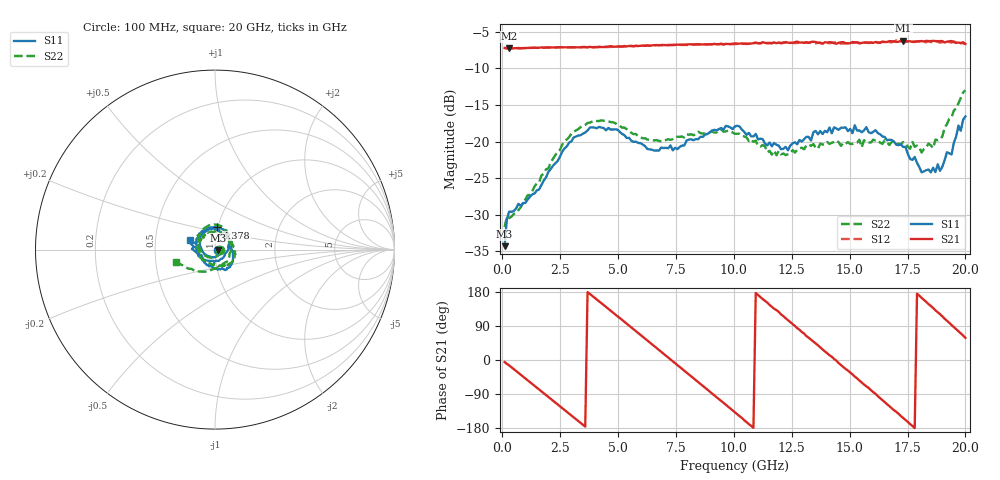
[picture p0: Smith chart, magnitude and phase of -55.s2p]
!Agilent Technologies,N5230C,MY49001569,A.09.33.09
!Agilent N5230C: A.09.33.09
!Date: Tuesday, July 28, 2015 16:40:22
!Correction: S11(Full 2 Port(1,2))
!S21(Full 2 Port(1,2))
!S12(Full 2 Port(1,2))
!S22(Full 2 Port(1,2))
!S2P File: Measurements: S11, S21, S12, S22:
# Hz S  dB  R 50
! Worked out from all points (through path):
!   201 points, 100 MHz to 20 GHz, reference 50 ohm
!   highest |S21| = -6.18 dB at 17.31 GHz (marker M1); lowest = -7.3 dB at 299 MHz (marker M2)
!   group delay of S21, straight-line fit = 141 ps
!   lowest |S11| = -34.3 dB at 100 MHz (marker M3), VSWR 1.04, Z = 52 - j0.208 ohm
!   |S11| at or under -10 dB: start of sweep to end of sweep
!   |S22| runs from -31.7 to -13.0 dB; largest |S21 - S12| = 0.02
!   S11 on the Smith chart (normalised r, x): 100 MHz: 1.04, -0.00; 4.378 GHz: 1.00, +0.25; 20 GHz: 0.75, +0.08
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1e8  -34.31 -6.0  -7.19 -5.3  -7.18 -4.8  -31.70 -5.9
2.99e8  -29.57 -18.7  -7.26 -14.4  -7.26 -14.7  -30.48 -21.7
1.891e9  -24.88 -148.2  -7.13 -92.8  -7.12 -92.6  -23.79 -148.7
3.483e9  -18.91 120.4  -7.05 -170.9  -7.09 -171.3  -17.80 124.0
4.3785e9  -18.13 83.7  -7.06 145.0  -7.06 144.8  -17.15 89.2
5.5725e9  -19.89 48.5  -6.94 86.0  -6.92 85.6  -18.80 52.2
6.7665e9  -21.24 19.5  -6.84 26.4  -6.81 26.2  -19.91 21.7
7.662e9  -20.73 0.2  -6.75 -18.3  -6.75 -18.7  -19.35 2.1
8.657e9  -19.35 -21.8  -6.72 -68.1  -6.70 -68.8  -18.90 -15.6
9.453e9  -18.14 -43.4  -6.60 -107.9  -6.67 -109.1  -18.34 -30.3
1.005e10  -17.91 -58.3  -6.57 -138.2  -6.66 -138.5  -18.93 -42.2
1.0846e10  -19.30 -80.5  -6.53 -178.8  -6.52 -179.0  -20.04 -63.9
1.1443e10  -20.52 -103.3  -6.52 151.6  -6.51 150.3  -21.46 -84.0
1.2438e10  -20.54 -152.2  -6.51 99.9  -6.47 99.1  -21.59 -125.4
1.3433e10  -18.72 162.1  -6.34 48.4  -6.54 47.9  -20.33 -167.8
1.47265e10  -18.11 124.7  -6.39 -18.3  -6.60 -18.3  -20.19 148.1
1.57215e10  -18.03 108.8  -6.44 -69.5  -6.45 -70.3  -20.16 127.1
1.67165e10  -19.74 66.5  -6.26 -121.6  -6.38 -122.2  -20.47 79.1
1.73135e10  -20.73 33.6  -6.18 -153.0  -6.28 -154.3  -20.06 42.7
1.81095e10  -24.20 -20.2  -6.24 164.1  -6.31 163.5  -21.50 -15.5
1.89055e10  -23.99 -99.2  -6.25 120.8  -6.48 118.9  -19.70 -87.5
2e10  -16.56 159.3  -6.65 58.4  -6.63 57.9  -12.97 -162.8
